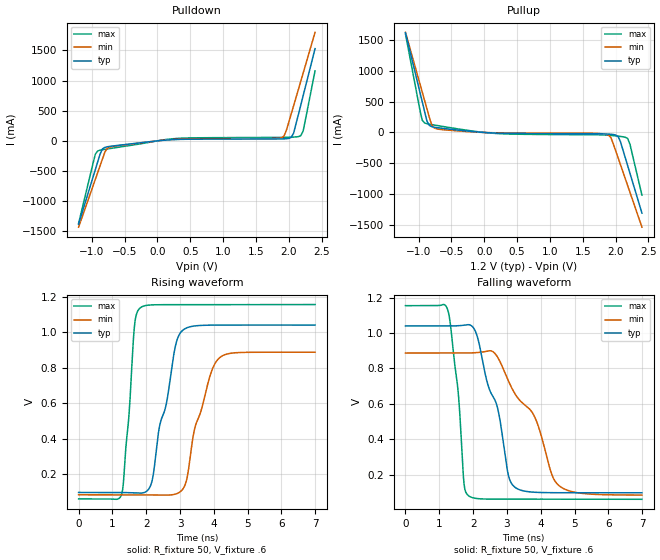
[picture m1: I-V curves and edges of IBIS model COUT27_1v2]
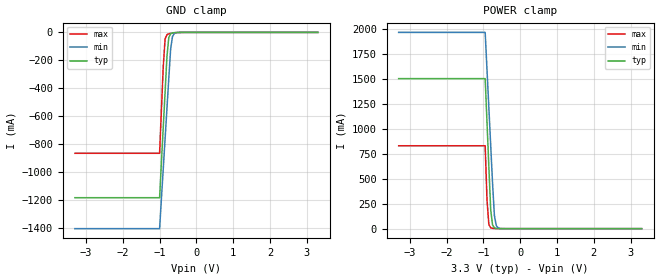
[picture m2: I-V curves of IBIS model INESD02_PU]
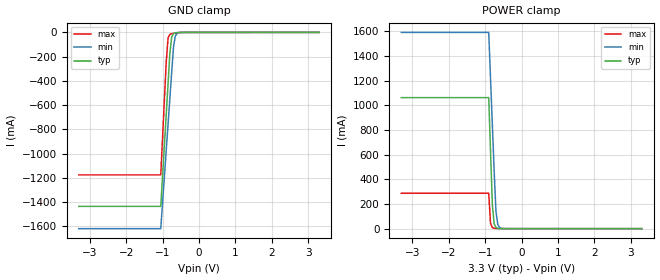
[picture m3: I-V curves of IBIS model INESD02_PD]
|   This file is an IBIS representation of the   |
|   Integrated Device Technology, Inc.   |
|   ICS8613   |
|   LOW SKEW, 1-TO-16, LVCMOS/LVTTL FANOUT BUFFER W/1.2V LVCMOS OUTPUTS   |
[IBIS Ver]   4.1
[File name]   8316_3v3_1v2.ibs
[File Rev]   1.0
[Date]   27 Mar 2009 | Last modified
|   May 22 2008  | Generated
[Source]   Originated at Integrated Devices Technology, Inc.
[Disclaimer]
IDT hereby grants the user of this IBIS model a non-exclusive,
nontransferable license to use this IBIS model under the following terms.
Before using this IBIS model, the user should read this license.
If the user does not accept these terms,  the IBIS model should be
returned to IDT within 30 days.
   The user is granted this license only to use the IBIS model and
is not granted rights to sell, load, rent, lease or license the IBIS
model in whole or in part, or in modified form to anyone other than
user. User may modify the IBIS model to suit its specific
applications but rights to derivative works and such modifications
shall belong to IDT.
   This IBIS model is provided on an "AS IS" basis and IDT makes
absolutely no warranty with respect to the information contained
herein. IDT DISCLAIMS AND CUSTOMER WAIVES ALL WARRANTIES, EXPRESS
OR IMPLIED, INCLUDING WARRANTIES OF MERCHANTABILITY OR FITNESS FOR
A PARTICULAR PURPOSE. The entire risk as to quality and performance
is with the Customer. ACCORDINGLY, IN NO EVENT SHALL THE COMPANY BE
LIABLE FOR ANY DAMAGES, WHETHER IN CONTRACT OR TORT,INCLUDING ANY
LOST PROFITS OR OTHER INCIDENTAL, CONSEQUENTIAL, EXEMPLARY, OR
PUNITIVE DAMAGES ARISING OUT OF THE USE OR APPLICATION OF THE IBIS
model provided in this package. Further, IDT reserves the right to
make changes without notice to any product herein to improve
reliability, function, or design. IDT does not convey any license
under patent rights or any other intellectual property rights,
including those of third parties.
   IDT is not obligated to provide maintenance or support
for the licensed IBIS model.
[Copyright]   Copyright 2008 by Integrated Device Technology, Inc.
[Component]   ICS8316K
[Manufacturer] Integrated Devices Technology, Inc.
[Package]
|QFN 32
|lead + wire   typ   min   max
R_pkg   72.4655m   58.886m   86.045m
L_pkg   1.47175nH   1.11650nH   1.77850nH
C_pkg   0.07747pF   0.07444pF   0.08050pF
[Pin] signal_name   model_name   R_pin   L_pin   C_pin
1   VDDO   POWER   86.045m   1.77850nH   0.08050pF
2   QA0   COUT27_1v2   76.996m   1.55783nH   0.07848pF
3   QA1   COUT27_1v2   67.941m   1.33717nH   0.07646pF
4   QA2   COUT27_1v2   58.886m   1.11650nH   0.07444pF
5   QA3   COUT27_1v2   58.886m   1.11650nH   0.07444pF
6   GND   GND   67.941m   1.33717nH   0.07646pF
7   OEA   INESD02_PU   76.996m   1.55783nH   0.07848pF
8   CLK   INESD02_PD   86.045m   1.77850nH   0.08050pF
9   VDD   POWER   86.045m   1.77850nH   0.08050pF
10   OEB   INESD02_PU   76.996m   1.55783nH   0.07848pF
11   GND   GND   67.941m   1.33717nH   0.07646pF
12   QB3   COUT27_1v2   58.886m   1.11650nH   0.07444pF
13   QB2   COUT27_1v2   58.886m   1.11650nH   0.07444pF
14   QB1   COUT27_1v2   67.941m   1.33717nH   0.07646pF
15   QB0   COUT27_1v2   76.996m   1.55783nH   0.07848pF
16   VDDO   POWER   86.045m   1.77850nH   0.08050pF
17   GND   GND   86.045m   1.77850nH   0.08050pF
18   OEC   INESD02_PU   76.996m   1.55783nH   0.07848pF
19   GND   GND   67.941m   1.33717nH   0.07646pF
20   QC3   COUT27_1v2   58.886m   1.11650nH   0.07444pF
21   QC2   COUT27_1v2   58.886m   1.11650nH   0.07444pF
22   QC1   COUT27_1v2   67.941m   1.33717nH   0.07646pF
23   QC0   COUT27_1v2   76.996m   1.55783nH   0.07848pF
24   VDDO   POWER   86.045m   1.77850nH   0.08050pF
25   VDDO   POWER   86.045m   1.77850nH   0.08050pF
26   QD0   COUT27_1v2   76.996m   1.55783nH   0.07848pF
27   QD1   COUT27_1v2   67.941m   1.33717nH   0.07646pF
28   QD2   COUT27_1v2   58.886m   1.11650nH   0.07444pF
29   QD3   COUT27_1v2   58.886m   1.11650nH   0.07444pF
30   GND   GND   67.941m   1.33717nH   0.07646pF
31   OED   INESD02_PU   76.996m   1.55783nH   0.07848pF
32   GND   GND   86.045m   1.77850nH   0.08050pF
| Models and submodels in the file (3): COUT27_1v2 (Output), INESD02_PU (Input), INESD02_PD (Input)
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[Model]   COUT27_1v2
|Model for buffer with 3.3V Core supply with 1.2V output supply
Model_type  Output
Polarity   Non-Inverting
Vmeas =.628V
Rref = 50
Cref = 0
Vref = .6V
|Variable  typ   min   max
C_comp   2p   1.5p   2.5p
[Voltage Range]   1.2V   1.14V   1.26V
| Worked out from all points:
|   slope of the pulldown table from 0 to 0.18 V, typ, clamps not added: 10.9 ohm
|   slope of the pullup table from 0 to 0.18 V, typ, clamps not added: 18.8 ohm
|   rising waveform, R_fixture 50, V_fixture .6: 20-80 % time 528ps typ, 581ps min, 242ps max; typ from 0.097 V to 1.04 V
|   falling waveform, R_fixture 50, V_fixture .6: 20-80 % time 691ps typ, 1.2ns min, 293ps max; typ from 1.04 V to 0.097 V
|  Voltage   I(typ)   I(min)   I(max)
[Pullup]
-1.2V     1.611A     1.617A     1.591A
-981.8mV  658mA      792.5mA    372.1mA
-945.5mV  499.2mA    655.1mA    199.4mA
-909.1mV  340.4mA    517.8mA    154.3mA
-836.4mV  114.3mA    243.3mA    133.9mA
-800mV    93.64mA    121.3mA    127.3mA
-727.3mV  79.24mA    58.81mA    114.3mA
218.2mV   -10.93mA   -5.847mA   -18.49mA
1.891V    -26.93mA   -43.43mA   -44.83mA
2.036V    -64.19mA   -406.2mA   -59.83mA
2.182V    -531.9mA   -854.7mA   -96.4mA
2.4V      -1.302A    -1.529A    -1.012A
|  Voltage   I(typ)   I(min)   I(max)
[Pulldown]
-1.2V     -1.382A    -1.432A    -1.368A
-945.5mV  -477.3mA   -639.2mA   -222.1mA
-836.4mV  -133.2mA   -299.2mA   -146.5mA
-800mV    -108.2mA   -186.6mA   -140.4mA
-727.3mV  -92.37mA   -105.4mA   -128.5mA
327.3mV   23.91mA    27.63mA    42.37mA
1.927V    33.48mA    80.7mA     57.73mA
2.036V    57.76mA    444.1mA    60.89mA
2.073V    124.7mA    579.2mA    62.8mA
2.182V    589.8mA    985.3mA    84.78mA
2.218V    746.1mA    1.121A     160.7mA
2.4V      1.53A      1.8A       1.161A
[Ramp]
|   typ   min   max
dV/dt_r   0.756/0.694n   0.643/0.802n   0.877/0.326n
dV/dt_f   0.759/0.885n   0.652/1.568n   0.880/0.393n
R_load =   50.0000
[Rising Waveform]
R_fixture = 50
V_fixture = .6   | VCC_typ
V_fixture_min = .57   | VCC_min
V_fixture_max = .63   | VCC_max
C_fixture = 0.0p
| Time   typ   min   max
0s        97.02mV    83.85mV    60.81mV
1.27ns    97.15mV    83.86mV    85.58mV
1.491ns   95.8mV     83.89mV    534.9mV
1.649ns   94.56mV    83.95mV    1.026V
1.817ns   93.35mV    83.86mV    1.135V
2.163ns   155mV      82.89mV    1.153V
2.846ns   905mV      86.92mV    1.154V
3.066ns   1.008V     112.4mV    1.154V
4.137ns   1.039V     849.6mV    1.154V
6.993ns   1.039V     886.6mV    1.155V
[Falling Waveform]
R_fixture = 50
V_fixture = .6   | VCC_typ
V_fixture_min = .57   | VCC_min
V_fixture_max = .63   | VCC_max
C_fixture = 0.0p
| Time   typ   min   max
0s        1.04V      886.6mV    1.154V
1.25ns    1.039V     886.5mV    1.13V
1.554ns   1.041V     886.4mV    675.7mV
1.732ns   1.044V     886.4mV    146.4mV
1.858ns   1.047V     886.6mV    81.15mV
2.615ns   632mV      889.9mV    60.96mV
3.203ns   133.7mV    667.9mV    60.82mV
3.811ns   100mV      529.3mV    60.81mV
4.547ns   97.2mV     136.4mV    60.81mV
6.993ns   97.06mV    84.03mV    59.92mV
[Model]   INESD02_PU
Model_type   Input
Polarity   Non-Inverting
Vinl = 0.80V
Vinh = 2.0V
|   typ   min   max
C_comp   2pF   1.5pF   2.5pF
|   typ   min   max
[Voltage range]  3.3V   3.15V   3.45V
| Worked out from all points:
|   GND clamp passes 1 mA (typ) near -0.56 V on its own axis
|   POWER clamp passes 1 mA (typ) near -0.61 V on its own axis
[GND_clamp]
|Voltage   I(typ)   I(min)   I(max)
-3.3V     -1.184A    -1.405A    -865.6mA
-1V       -1.184A    -1.405A    -865.6mA
-900mV    -678.5mA   -975.1mA   -244.1mA
-850mV    -426.2mA   -760.2mA   -46.92mA
-800mV    -174mA     -545.4mA   -16.17mA
-750mV    -37.03mA   -330.8mA   -9.981mA
-700mV    -9.767mA   -120.3mA   -7.122mA
-650mV    -3.616mA   -29.78mA   -4.922mA
-600mV    -1.7mA     -7.594mA   -3.115mA
-400mV    -123.9uA   -126uA     -173.9uA
3.3V      1.866nA    3.949uA    0A
[POWER_clamp]
|Voltage   I(typ)   I(min)   I(max)
-3.3V     1.506A     1.97A      832.1mA
-950mV    1.506A     1.97A      832.1mA
-900mV    1.063A     1.592A     287.2mA
-850mV    620.4mA    1.215A     41.77mA
-800mV    191.5mA    837.4mA    8.692mA
-750mV    37.69mA    460.1mA    3.262mA
-700mV    8.032mA    133.8mA    1.662mA
-650mV    2.005mA    32.58mA    840.1uA
-600mV    607uA      8.009mA    378.6uA
-450mV    33.11uA    139.8uA    23.88uA
3.3V      -71.13uA   -77.46uA   -62.11uA
[Model]   INESD02_PD
Model_type   Input
Polarity   Non-Inverting
Vinl = 0.80V
Vinh = 2.0V
|   typ   min   max
C_comp   2pF   1.5pF   2.5pF
|   typ   min   max
[Voltage range]  3.3V   3.15V   3.45V
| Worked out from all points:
|   GND clamp passes 1 mA (typ) near -0.56 V on its own axis
|   POWER clamp passes 1 mA (typ) near -0.61 V on its own axis
[GND_clamp]
|Voltage   I(typ)   I(min)   I(max)
-3.3V     -1.436A    -1.62A     -1.176A
-1.05V    -1.436A    -1.62A     -1.176A
-900mV    -678.5mA   -975.1mA   -244mA
-850mV    -426.1mA   -760.1mA   -46.85mA
-800mV    -173.9mA   -545.4mA   -16.11mA
-750mV    -36.96mA   -330.7mA   -9.916mA
-700mV    -9.696mA   -120.2mA   -7.056mA
-650mV    -3.545mA   -29.7mA    -4.857mA
-600mV    -1.629mA   -7.52mA    -3.049mA
-400mV    -52.81uA   -52.52uA   -108.7uA
3.3V      71.13uA    77.43uA    62.11uA
[POWER_clamp]
|Voltage   I(typ)   I(min)   I(max)
-3.3V     1.063A     1.593A     287.3mA
-900mV    1.063A     1.593A     287.3mA
-850mV    620.5mA    1.215A     41.84mA
-800mV    191.6mA    837.5mA    8.757mA
-750mV    37.76mA    460.2mA    3.328mA
-700mV    8.104mA    133.8mA    1.728mA
-650mV    2.076mA    32.66mA    905.3uA
-600mV    678.1uA    8.083mA    443.8uA
-450mV    104.2uA    213.3uA    89.09uA
3.3V      -3.041nA   -3.986uA   0A
